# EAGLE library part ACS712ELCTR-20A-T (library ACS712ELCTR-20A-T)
Linear Current Sensor
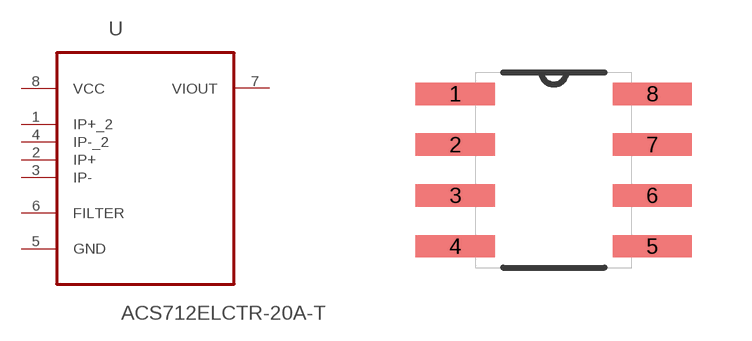
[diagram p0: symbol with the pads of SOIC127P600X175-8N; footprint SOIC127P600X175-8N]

Designator prefix U

## ACS712ELCTR-20A-T (Availability: Good; Description: Fully Integrated, Hall Effect-Based Linear Current Sensor IC with 2.1 kVRMS Voltage Isolation and a Low-Resistance Cu...; MF: Allegro MicroSystems LLC; MP: ACS712ELCTR-20A-T; Package: SOIC-8 Allegro MicroSystems LLC; Price: 2.80 USD)  [SOIC127P600X175-8N]
1  IP+_2  in
2  IP+  in
3  IP-  in
4  IP-_2  in
5  GND  pas
6  FILTER  in
7  VIOUT  out
8  VCC  pwr

## Footprint SOIC127P600X175-8N (pad centres in mm)
smd 1.981 x 0.559: 1 -2.464,1.905; 2 -2.464,0.635; 3 -2.464,-0.635; 4 -2.464,-1.905; 5 2.464,-1.905; 6 2.464,-0.635; 7 2.464,0.635; 8 2.464,1.905

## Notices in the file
This work is licensed under a Creative Commons Attribution-ShareAlike 4.0 International License (CC BY-SA) with Design Exception 1.0
